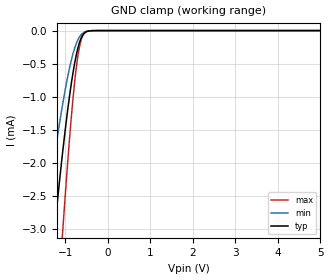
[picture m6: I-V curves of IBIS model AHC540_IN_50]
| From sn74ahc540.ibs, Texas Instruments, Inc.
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[Model]   AHC540_IN_50
Model_type  Input
Vinl = 1.65
Vinh = 3.85
| variable   typ   min   max
C_comp   0.58pF   0.52pF   0.65pF
[Temperature Range]   40   100   -40
| Ambient temperature   25   85   -40
[Voltage range]   5   4.5   5.5
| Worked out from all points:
|   GND clamp passes 1 mA (typ) near -0.91 V on its own axis
[GND Clamp]
| AHC540_IN_50
|   Voltage   I(typ)   I(min)   I(max)
-5V       -39.52mA   -26.01mA   -50.56mA
-1.5V     -4.735mA   -3.021mA   -7.495mA
-1.27V    -3.109mA   -1.953mA   -5.058mA
-1.245V   -2.945mA   -1.844mA   -4.802mA
-1.07V    -1.866mA   -1.133mA   -3.091mA
-1.05V    -1.752mA   -1.058mA   -2.905mA
-875mV    -861.9uA   -485.8uA   -1.416mA
-765mV    -434.8uA   -232.8uA   -674.8uA
-665mV    -173.4uA   -93.49uA   -235.2uA
-615mV    -93.71uA   -53.16uA   -114.8uA
-545mV    -32.8uA    -20.51uA   -33.5uA
5V        15.07nA    1.006nA    138.2nA
